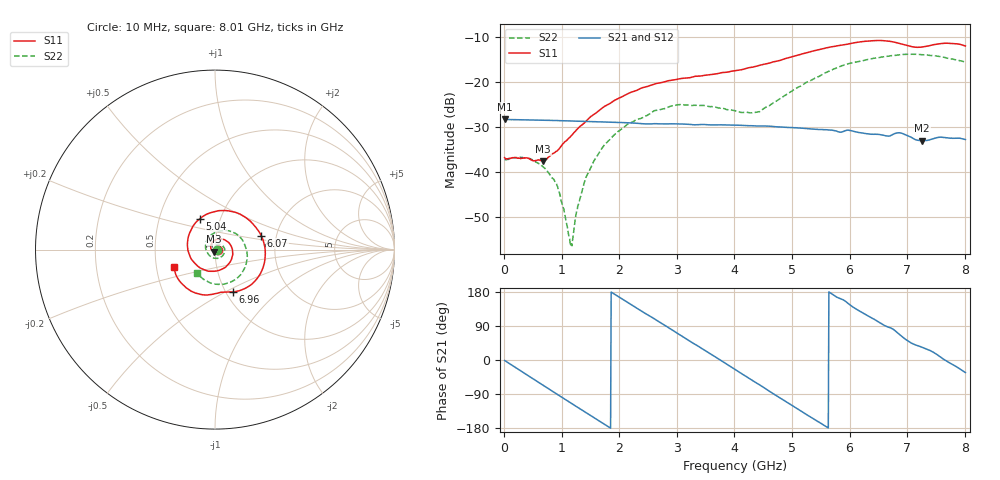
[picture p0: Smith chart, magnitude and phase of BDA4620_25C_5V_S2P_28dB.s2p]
!Agilent Technologies,E5071B,MY42404982,A.09.10
!Date: Wed May 06 09:04:34 2026
!Data & Calibration Information:
!Freq	S11:SOLT2(ON)	S21:SOLT2(ON)	S12:SOLT2(ON)	S22:SOLT2(ON)
# Hz S RI R 50
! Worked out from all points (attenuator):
!   801 points, 10 MHz to 8.01 GHz, reference 50 ohm
!   highest |S21| = -28.38 dB at 10 MHz (marker M1); lowest = -33.1 dB at 7.26 GHz (marker M2)
!   lowest |S11| = -37.7 dB at 680 MHz (marker M3), VSWR 1.03, Z = 49.6 - j1.23 ohm
!   |S11| at or under -10 dB: start of sweep to end of sweep
!   |S22| runs from -56.6 to -13.9 dB; largest |S21 - S12| = 0.00017
!   S11 on the Smith chart (normalised r, x): 10 MHz: 1.03, -0.00; 5.04 GHz: 0.80, +0.29; 6.07 GHz: 1.66, +0.28; 6.96 GHz: 1.08, -0.54; 8.01 GHz: 0.62, -0.13
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1e7  0.0142 -0.00097  0.0381 -0.000828  0.0381 -0.000802  0.0135 -0.000437
4.2e8  0.00748 -0.0119  0.0282 -0.0248  0.0282 -0.0249  0.0133 -0.00465
6.8e8  -0.0039 -0.0124  0.0147 -0.0342  0.0147 -0.0343  0.00919 -0.00651
9.3e8  -0.0163 -0.00523  -0.000742 -0.0369  -0.000764 -0.037  0.00356 -0.00582
1.16e9  -0.023 0.00893  -0.0146 -0.0335  -0.0146 -0.0336  -0.00129 -0.000734
1.19e9  -0.0235 0.0112  -0.0162 -0.0327  -0.0163 -0.0328  -0.00174 5.64e-05
1.35e9  -0.0229 0.0237  -0.0242 -0.027  -0.0242 -0.027  -0.00329 0.00489
1.53e9  -0.0164 0.0385  -0.0309 -0.0185  -0.0309 -0.0185  -0.00304 0.0115
1.77e9  0.0018 0.054  -0.0352 -0.00485  -0.0353 -0.00485  0.00112 0.0205
2.15e9  0.0457 0.0574  -0.0306 0.0168  -0.0306 0.0168  0.0173 0.029
2.68e9  0.0962 0.00448  -0.00697 0.0333  -0.00699 0.0333  0.0443 0.0192
3.08e9  0.0876 -0.0637  0.0149 0.0303  0.0151 0.0303  0.055 -0.00752
4.01e9  -0.0904 -0.0968  0.0298 -0.0138  0.0298 -0.0138  -0.0107 -0.0463
4.43e9  -0.1514 -0.000404  0.0136 -0.0291  0.0136 -0.0292  -0.0448 -0.0114
5.04e9  -0.0834 0.1726  -0.0171 -0.0256  -0.0172 -0.0256  -0.0264 0.0771
5.35e9  0.0198 0.2167  -0.0265 -0.0135  -0.0266 -0.0135  0.0231 0.1022
6.07e9  0.2577 0.078  -0.021 0.0186  -0.0211 0.0186  0.156 0.0478
6.68e9  0.2065 -0.191  0.00158 0.0248  0.00157 0.0248  0.1696 -0.0896
6.96e9  0.0989 -0.2353  0.0145 0.0213  0.0146 0.0214  0.1329 -0.1502
7.26e9  0.0182 -0.2416  0.0185 0.0121  0.0185 0.0122  0.0636 -0.1886
7.63e9  -0.1203 -0.2374  0.024 0.000915  0.024 0.000985  -0.0284 -0.1848
8.01e9  -0.228 -0.0993  0.019 -0.0124  0.0191 -0.0124  -0.1027 -0.1283
